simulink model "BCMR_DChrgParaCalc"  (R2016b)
settings: Solver=FixedStepDiscrete  StartTime=0.0  StopTime=10  FixedStep=0.01  RelTol=1e-3  EnableMultiTasking=on
undefined symbols (not defined in the file or in its folder): BCMR_ahDChgBattNominalCapa_C, BCMR_bCurrCalSelect_C, BCMR_bCurrIncDeltaLimEna_C, BCMR_bDChrgFulChkTenEna_C, BCMR_bDChrgFulChkThreeEna_C, BCMR_cntCoolDFC_CW, BCMR_cntSoh_CW, BCMR_G1E0PlatformSwPara_C, BCMR_iCurrDcr_C, BCMR_iDcChrgCurrAbnorm_T, BCMR_iDcChrgCurrAbnormMAP_T, BCMR_iDcChrgCurrNew_T, BCMR_iDcChrgCurrNewMAP_T, BCMR_iDcChrgCurrOld_T, BCMR_iDcChrgCurrOldAbnorm_T, BCMR_iDcChrgCurrOldAbnormMAP_T, BCMR_iDcChrgCurrOldMAP_T, BCMR_iDCCurrDecStep_C, BCMR_iDCCurrDecThrd_C, BCMR_iDCCurrDeltaLim_C, BCMR_iDCCurrDiff_C, BCMR_iDCCurrFil_C, BCMR_iDCCurrIncStep_C, BCMR_iDCCurrIncThrd_C, BCMR_iDChrgCurrCutOff_C, BCMR_kmAcmDist_C, BCMR_numCcsPwrSelc_C, BCMR_numCellVoltFull_C, BCMR_numCellVoltFullThree_C, BCMR_numCurrCalcEna, BCMR_pCcsPwrSelc_C, BCMR_pctBmsPwrRdc_C, BCMR_rCurrDcr_C, BCMR_rCurrIcr_C, BCMR_rDchrgLoadCoef_C, BCMR_tBattTempMaxFil_C, BCMR_tBattTempSelcLmtDwn_C, BCMR_tBattTempSelcLmtUp_C, BCMR_tDcChrgCellTemp1_A, BCMR_tDcChrgCellTemp2_A, BCMR_tDcChrgCellTemp_A, BCMR_tDchrgLoadLmt_C, BCMR_tiBattTempMaxFilDly_C, BCMR_tiBattTempSwitch_C, BCMR_tiCellVoltFullCnt_C, BCMR_tiCellVoltMaxFilDly_C, BCMR_tiCurrHysTimeDelay_C, BCMR_tiDcChrgPwrCCSDebs_C, BCMR_tiDChgFullPreHold_C, BCMR_tiDChrgCurrReqCalDly_C, BCMR_tiDChrgDetParaDebs_C, BCMR_tiDChrgFullBase_C, BCMR_tiDChrgFullDebs_C, BCMR_tiDChrgFulParaDebs_C, BCMR_tiDChrgFulWait_C, BCMR_tiDChrgParaBase_C, BCMR_tiHoldOnToCurrCalcOff_C, BCMR_tTempDisMapX_A, BCMR_tTempDisMapY_A, BCMR_uBattVoltOff_C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
libraries: simulink x34
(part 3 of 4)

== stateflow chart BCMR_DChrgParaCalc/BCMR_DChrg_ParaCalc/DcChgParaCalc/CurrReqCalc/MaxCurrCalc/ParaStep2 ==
  state Init
    en:
    ParaStep = 0;
  state ParaStep1
    en:
    ParaStep = BCMR_ParaStep_A[0];
  state ParaStep2
    en:
    ParaStep = BCMR_ParaStep_A[1];
  state ParaStep3
    en:
    ParaStep = BCMR_ParaStep_A[2];
  state ParaStep4
    en:
    ParaStep = BCMR_ParaStep_A[3];
  state ParaStep5
    en:
    ParaStep = BCMR_ParaStep_A[4];
  state ParaStep6
    en:
    ParaStep = BCMR_ParaStep_A[5];
  state ParaStep7
    en:
    ParaStep = BCMR_ParaStep_A[6];
  state ParaStep8
    en:
    ParaStep = BCMR_ParaStep_A[7];
  state ParaStep9
    en:
    ParaStep = BCMR_ParaStep_A[8];
  state ParaStep10
    en:
    ParaStep = BCMR_ParaStep_A[9];
  state ParaStep11
    en:
    ParaStep = BCMR_ParaStep_A[10];
  state ParaStep12
    en:
    ParaStep = BCMR_ParaStep_A[11];
  state ParaStep13
    en:
    ParaStep = BCMR_ParaStep_A[12];
  state ParaStep14
    en:
    ParaStep = BCMR_ParaStep_A[13];
  (default) -> Init
  Init -> (junction 26) : [BattTemp >= BCMR_BattPara_A[0]]
  (junction 488) -> Init
  (junction 26) -> (junction 27)
  (junction 489) -> (junction 488)
  Init -> ParaStep1 : [BattTemp < BCMR_BattPara_A[0]]
  (junction 453) -> ParaStep1
  (junction 456) -> (junction 453)
  ParaStep1 -> ParaStep2 : [BattTemp >= BCMR_BattPara_A[0] ]
  ParaStep2 -> (junction 456) : [BattTemp < BCMR_BattPara_A[0] ]
  (junction 27) -> ParaStep2
  (junction 447) -> (junction 456)
  (junction 27) -> (junction 28) : [BattTemp >= BCMR_BattPara_A[1] ]
  (junction 450) -> ParaStep2
  ParaStep2 -> ParaStep3 : [BattTemp >= BCMR_BattPara_A[1] ]
  (junction 444) -> (junction 450)
  (junction 28) -> ParaStep3
  ParaStep3 -> (junction 444) : [BattTemp < BCMR_BattPara_A[1] - BCMR_HysRng_C]
  (junction 444) -> (junction 447) : [BattTemp < BCMR_BattPara_A[0] ]
  (junction 28) -> (junction 29) : [BattTemp >= BCMR_BattPara_A[2] ]
  (junction 430) -> (junction 444)
  (junction 431) -> (junction 447)
  (junction 441) -> ParaStep3
  (junction 426) -> (junction 441)
  ParaStep3 -> ParaStep4 : [BattTemp >= BCMR_BattPara_A[2] ]
  ParaStep4 -> (junction 426) : [BattTemp < BCMR_BattPara_A[2] - BCMR_HysRng_C]
  (junction 426) -> (junction 430) : [BattTemp < BCMR_BattPara_A[1] - BCMR_HysRng_C]
  (junction 430) -> (junction 431) : [BattTemp < BCMR_BattPara_A[0] ]
  (junction 472) -> (junction 426)
  (junction 473) -> (junction 430)
  (junction 475) -> (junction 431)
  (junction 29) -> ParaStep4
  (junction 29) -> (junction 30) : [BattTemp >= BCMR_BattPara_A[3]]
  (junction 423) -> ParaStep4
  (junction 474) -> (junction 423)
  ParaStep4 -> ParaStep5 : [BattTemp >= BCMR_BattPara_A[3]]
  ParaStep5 -> (junction 474) : [BattTemp < BCMR_BattPara_A[3] - BCMR_HysRng_C]
  (junction 474) -> (junction 472) : [BattTemp < BCMR_BattPara_A[2] - BCMR_HysRng_C]
  (junction 472) -> (junction 473) : [BattTemp < BCMR_BattPara_A[1] - BCMR_HysRng_C]
  (junction 473) -> (junction 475) : [BattTemp < BCMR_BattPara_A[0] ]
  (junction 30) -> ParaStep5
  (junction 401) -> (junction 474)
  (junction 389) -> (junction 472)
  (junction 400) -> (junction 473)
  (junction 398) -> (junction 475)
  (junction 30) -> (junction 31) : [BattTemp >= BCMR_BattPara_A[4] ]
  (junction 408) -> ParaStep5
  (junction 392) -> (junction 408)
  ParaStep5 -> ParaStep6 : [BattTemp >= BCMR_BattPara_A[4] ]
  ParaStep6 -> (junction 392) : [BattTemp < BCMR_BattPara_A[4] - BCMR_HysRng_C]
  (junction 392) -> (junction 401) : [BattTemp < BCMR_BattPara_A[3] - BCMR_HysRng_C]
  (junction 401) -> (junction 389) : [BattTemp < BCMR_BattPara_A[2] - BCMR_HysRng_C]
  (junction 389) -> (junction 400) : [BattTemp < BCMR_BattPara_A[1] - BCMR_HysRng_C]
  (junction 400) -> (junction 398) : [BattTemp < BCMR_BattPara_A[0] ]
  (junction 375) -> (junction 392)
  (junction 371) -> (junction 401)
  (junction 364) -> (junction 389)
  (junction 369) -> (junction 400)
  (junction 376) -> (junction 398)
  (junction 31) -> ParaStep6
  (junction 31) -> (junction 74) : [BattTemp >= BCMR_BattPara_A[5] ]
  (junction 384) -> ParaStep6
  (junction 373) -> (junction 384)
  ParaStep6 -> ParaStep7 : [BattTemp >= BCMR_BattPara_A[5] ]
  ParaStep7 -> (junction 373) : [BattTemp < BCMR_BattPara_A[5] - BCMR_HysRng_C]
  (junction 373) -> (junction 375) : [BattTemp < BCMR_BattPara_A[4] - BCMR_HysRng_C]
  (junction 375) -> (junction 371) : [BattTemp < BCMR_BattPara_A[3] - BCMR_HysRng_C]
  (junction 371) -> (junction 364) : [BattTemp < BCMR_BattPara_A[2] - BCMR_HysRng_C]
  (junction 364) -> (junction 369) : [BattTemp < BCMR_BattPara_A[1] - BCMR_HysRng_C]
  (junction 369) -> (junction 376) : [BattTemp < BCMR_BattPara_A[0]]
  (junction 341) -> (junction 373)
  (junction 349) -> (junction 375)
  (junction 352) -> (junction 371)
  (junction 343) -> (junction 364)
  (junction 353) -> (junction 369)
  (junction 350) -> (junction 376)
  (junction 74) -> ParaStep7
  (junction 74) -> (junction 75) : [BattTemp >= BCMR_BattPara_A[6] ]
  (junction 169) -> ParaStep7
  (junction 337) -> (junction 169)
  ParaStep7 -> ParaStep8 : [BattTemp >= BCMR_BattPara_A[6] ]
  ParaStep8 -> (junction 337) : [BattTemp < BCMR_BattPara_A[6] - BCMR_HysRng_C]
  (junction 337) -> (junction 341) : [BattTemp < BCMR_BattPara_A[5] - BCMR_HysRng_C]
  (junction 341) -> (junction 349) : [BattTemp < BCMR_BattPara_A[4] - BCMR_HysRng_C]
  (junction 349) -> (junction 352) : [BattTemp < BCMR_BattPara_A[3] - BCMR_HysRng_C]
  (junction 352) -> (junction 343) : [BattTemp < BCMR_BattPara_A[2] - BCMR_HysRng_C]
  (junction 343) -> (junction 353) : [BattTemp < BCMR_BattPara_A[1] - BCMR_HysRng_C]
  (junction 353) -> (junction 350) : [BattTemp < BCMR_BattPara_A[0] ]
  (junction 75) -> ParaStep8
  (junction 313) -> (junction 337)
  (junction 321) -> (junction 341)
  (junction 328) -> (junction 349)
  (junction 331) -> (junction 352)
  (junction 319) -> (junction 343)
  (junction 334) -> (junction 353)
  (junction 330) -> (junction 350)
  (junction 75) -> (junction 76) : [BattTemp >= BCMR_BattPara_A[7] ]
  (junction 148) -> ParaStep8
  (junction 310) -> (junction 148)
  ParaStep8 -> ParaStep9 : [BattTemp >= BCMR_BattPara_A[7] ]
  ParaStep9 -> (junction 310) : [BattTemp < BCMR_BattPara_A[7] - BCMR_HysRng_C]
  (junction 310) -> (junction 313) : [BattTemp < BCMR_BattPara_A[6] - BCMR_HysRng_C]
  (junction 313) -> (junction 321) : [BattTemp < BCMR_BattPara_A[5] - BCMR_HysRng_C]
  (junction 321) -> (junction 328) : [BattTemp < BCMR_BattPara_A[4] - BCMR_HysRng_C]
  (junction 328) -> (junction 331) : [BattTemp < BCMR_BattPara_A[3] - BCMR_HysRng_C]
  (junction 331) -> (junction 319) : [BattTemp < BCMR_BattPara_A[2] - BCMR_HysRng_C]
  (junction 319) -> (junction 334) : [BattTemp < BCMR_BattPara_A[1] - BCMR_HysRng_C]
  (junction 334) -> (junction 330) : [BattTemp < BCMR_BattPara_A[0]]
  (junction 280) -> (junction 310)
  (junction 283) -> (junction 313)
  (junction 299) -> (junction 321)
  (junction 295) -> (junction 328)
  (junction 293) -> (junction 331)
  (junction 287) -> (junction 319)
  (junction 290) -> (junction 334)
  (junction 292) -> (junction 330)
  (junction 76) -> ParaStep9
  (junction 76) -> (junction 77) : [BattTemp >= BCMR_BattPara_A[8] ]
  (junction 140) -> ParaStep9
  (junction 277) -> (junction 140)
  ParaStep9 -> ParaStep10 : [BattTemp >= BCMR_BattPara_A[8] ]
  ParaStep10 -> (junction 277) : [BattTemp < BCMR_BattPara_A[8] - BCMR_HysRng_C]
  (junction 277) -> (junction 280) : [BattTemp < BCMR_BattPara_A[7] - BCMR_HysRng_C]
  (junction 280) -> (junction 283) : [BattTemp < BCMR_BattPara_A[6] - BCMR_HysRng_C]
  (junction 283) -> (junction 299) : [BattTemp < BCMR_BattPara_A[5] - BCMR_HysRng_C]
  (junction 299) -> (junction 295) : [BattTemp < BCMR_BattPara_A[4] - BCMR_HysRng_C]
  (junction 295) -> (junction 293) : [BattTemp < BCMR_BattPara_A[3] - BCMR_HysRng_C]
  (junction 293) -> (junction 287) : [BattTemp < BCMR_BattPara_A[2] - BCMR_HysRng_C]
  (junction 287) -> (junction 290) : [BattTemp < BCMR_BattPara_A[1] - BCMR_HysRng_C]
  (junction 290) -> (junction 292) : [BattTemp < BCMR_BattPara_A[0] ]
  (junction 228) -> (junction 277)
  (junction 230) -> (junction 280)
  (junction 232) -> (junction 283)
  (junction 247) -> (junction 299)
  (junction 253) -> (junction 295)
  (junction 249) -> (junction 293)
  (junction 259) -> (junction 287)
  (junction 256) -> (junction 290)
  (junction 246) -> (junction 292)
  (junction 77) -> ParaStep10
  (junction 77) -> (junction 78) : [BattTemp >= BCMR_BattPara_A[9] ]
  (junction 132) -> ParaStep10
  (junction 226) -> (junction 132)
  ParaStep10 -> ParaStep11 : [BattTemp >= BCMR_BattPara_A[9] ]
  ParaStep11 -> (junction 226) : [BattTemp < BCMR_BattPara_A[9] - BCMR_HysRng_C]
  (junction 226) -> (junction 228) : [BattTemp < BCMR_BattPara_A[8] - BCMR_HysRng_C]
  (junction 228) -> (junction 230) : [BattTemp < BCMR_BattPara_A[7] - BCMR_HysRng_C]
  (junction 230) -> (junction 232) : [BattTemp < BCMR_BattPara_A[6] - BCMR_HysRng_C]
  (junction 232) -> (junction 247) : [BattTemp < BCMR_BattPara_A[5] - BCMR_HysRng_C]
  (junction 247) -> (junction 253) : [BattTemp < BCMR_BattPara_A[4] - BCMR_HysRng_C]
  (junction 253) -> (junction 249) : [BattTemp < BCMR_BattPara_A[3] - BCMR_HysRng_C]
  (junction 249) -> (junction 259) : [BattTemp < BCMR_BattPara_A[2] - BCMR_HysRng_C]
  (junction 259) -> (junction 256) : [BattTemp < BCMR_BattPara_A[1] - BCMR_HysRng_C]
  (junction 256) -> (junction 246) : [BattTemp < BCMR_BattPara_A[0] ]
  (junction 78) -> ParaStep11
  (junction 196) -> (junction 226)
  (junction 199) -> (junction 228)
  (junction 202) -> (junction 230)
  (junction 205) -> (junction 232)
  (junction 213) -> (junction 247)
  (junction 210) -> (junction 253)
  (junction 211) -> (junction 249)
  (junction 212) -> (junction 259)
  (junction 222) -> (junction 256)
  (junction 220) -> (junction 246)
  (junction 78) -> (junction 79) : [BattTemp >= BCMR_BattPara_A[10]]
  (junction 127) -> ParaStep11
  (junction 241) -> (junction 127)
  ParaStep11 -> ParaStep12 : [BattTemp >= BCMR_BattPara_A[10]]
  ParaStep12 -> (junction 241) : [BattTemp < BCMR_BattPara_A[10] - BCMR_HysRng_C]
  (junction 241) -> (junction 196) : [BattTemp < BCMR_BattPara_A[9] - BCMR_HysRng_C]
  (junction 196) -> (junction 199) : [BattTemp < BCMR_BattPara_A[8] - BCMR_HysRng_C]
  (junction 199) -> (junction 202) : [BattTemp < BCMR_BattPara_A[7] - BCMR_HysRng_C]
  (junction 202) -> (junction 205) : [BattTemp < BCMR_BattPara_A[6] - BCMR_HysRng_C]
  (junction 205) -> (junction 213) : [BattTemp < BCMR_BattPara_A[5] - BCMR_HysRng_C]
  (junction 213) -> (junction 210) : [BattTemp < BCMR_BattPara_A[4] - BCMR_HysRng_C]
  (junction 210) -> (junction 211) : [BattTemp < BCMR_BattPara_A[3] - BCMR_HysRng_C]
  (junction 211) -> (junction 212) : [BattTemp < BCMR_BattPara_A[2] - BCMR_HysRng_C]
  (junction 212) -> (junction 222) : [BattTemp < BCMR_BattPara_A[1] - BCMR_HysRng_C]
  (junction 222) -> (junction 220) : [BattTemp < BCMR_BattPara_A[0] ]
  (junction 79) -> ParaStep12
  (junction 124) -> (junction 241)
  (junction 135) -> (junction 196)
  (junction 143) -> (junction 199)
  (junction 151) -> (junction 202)
  (junction 154) -> (junction 205)
  (junction 156) -> (junction 213)
  (junction 157) -> (junction 210)
  (junction 158) -> (junction 211)
  (junction 159) -> (junction 212)
  (junction 164) -> (junction 222)
  (junction 166) -> (junction 220)
  (junction 79) -> (junction 80) : [BattTemp >= BCMR_BattPara_A[11] ]
  (junction 119) -> ParaStep12
  (junction 238) -> (junction 119)
  ParaStep12 -> ParaStep13 : [BattTemp >= BCMR_BattPara_A[11] ]
  (junction 80) -> ParaStep13
  ParaStep13 -> (junction 238) : [BattTemp < BCMR_BattPara_A[11] - BCMR_HysRng_C]
  (junction 238) -> (junction 124) : [BattTemp < BCMR_BattPara_A[10] - BCMR_HysRng_C]
  (junction 124) -> (junction 135) : [BattTemp < BCMR_BattPara_A[9] - BCMR_HysRng_C]
  (junction 135) -> (junction 143) : [BattTemp < BCMR_BattPara_A[8] - BCMR_HysRng_C]
  (junction 143) -> (junction 151) : [BattTemp < BCMR_BattPara_A[7] - BCMR_HysRng_C]
  (junction 151) -> (junction 154) : [BattTemp < BCMR_BattPara_A[6] - BCMR_HysRng_C]
  (junction 154) -> (junction 156) : [BattTemp < BCMR_BattPara_A[5] - BCMR_HysRng_C]
  (junction 156) -> (junction 157) : [BattTemp < BCMR_BattPara_A[4] - BCMR_HysRng_C]
  (junction 157) -> (junction 158) : [BattTemp < BCMR_BattPara_A[3] - BCMR_HysRng_C]
  (junction 158) -> (junction 159) : [BattTemp < BCMR_BattPara_A[2] - BCMR_HysRng_C]
  (junction 159) -> (junction 164) : [BattTemp < BCMR_BattPara_A[1] - BCMR_HysRng_C]
  (junction 164) -> (junction 166) : [BattTemp < BCMR_BattPara_A[0] ]
  (junction 80) -> (junction 81) : [BattTemp >= BCMR_BattPara_A[12] ]
  (junction 115) -> (junction 238)
  (junction 117) -> (junction 124)
  (junction 130) -> (junction 135)
  (junction 138) -> (junction 143)
  (junction 146) -> (junction 151)
  (junction 181) -> (junction 154)
  (junction 179) -> (junction 156)
  (junction 176) -> (junction 157)
  (junction 177) -> (junction 158)
  (junction 178) -> (junction 159)
  (junction 185) -> (junction 164)
  (junction 184) -> (junction 166)
  (junction 462) -> ParaStep13
  (junction 460) -> (junction 462)
  ParaStep13 -> ParaStep14 : [BattTemp >= BCMR_BattPara_A[12] ]
  (junction 81) -> ParaStep14
  ParaStep14 -> (junction 460) : [BattTemp < BCMR_BattPara_A[12] - BCMR_HysRng_C]
  (junction 460) -> (junction 115) : [BattTemp < BCMR_BattPara_A[11] - BCMR_HysRng_C]
  (junction 115) -> (junction 117) : [BattTemp < BCMR_BattPara_A[10] - BCMR_HysRng_C]
  (junction 117) -> (junction 130) : [BattTemp < BCMR_BattPara_A[9] - BCMR_HysRng_C]
  (junction 130) -> (junction 138) : [BattTemp < BCMR_BattPara_A[8] - BCMR_HysRng_C]
  (junction 138) -> (junction 146) : [BattTemp < BCMR_BattPara_A[7] - BCMR_HysRng_C]
  (junction 146) -> (junction 181) : [BattTemp < BCMR_BattPara_A[6] - BCMR_HysRng_C]
  (junction 181) -> (junction 179) : [BattTemp < BCMR_BattPara_A[5] - BCMR_HysRng_C]
  (junction 179) -> (junction 176) : [BattTemp < BCMR_BattPara_A[4] - BCMR_HysRng_C]
  (junction 176) -> (junction 177) : [BattTemp < BCMR_BattPara_A[3] - BCMR_HysRng_C]
  (junction 177) -> (junction 178) : [BattTemp < BCMR_BattPara_A[2] - BCMR_HysRng_C]
  (junction 178) -> (junction 185) : [BattTemp < BCMR_BattPara_A[1] - BCMR_HysRng_C]
  (junction 185) -> (junction 184) : [BattTemp < BCMR_BattPara_A[0] ]
  (junction 81) -> (junction 467) : [BattTemp >= BCMR_BattPara_A[13] ]
  ParaStep14 -> (junction 493) : [BattTemp >= BCMR_BattPara_A[13] ]
  (junction 467) -> (junction 493)
  (junction 493) -> (junction 489)
  data: BattTemp input single; ParaStep output uint8; BCMR_BattPara_A input single; BCMR_ParaStep_A input uint8; BCMR_HysRng_C input single

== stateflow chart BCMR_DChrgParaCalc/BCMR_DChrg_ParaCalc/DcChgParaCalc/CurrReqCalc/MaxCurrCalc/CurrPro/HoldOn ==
  state Init
    en:
    CurrMethod = uint8(0);
  state HoldOn
    en:
    StepKeepL = VoltStepLast;
    StepKeepN = VoltStepNext;
    TempKeepL = TempStepL;
    TempKeepN = TempStep;
    CurrMethod = uint8(1);
  state CurrCalc
    state Init
      (default) -> (junction 296) : {CurrMethod = uint8(3);}
      (junction 296) -> (junction 297) : [FirstFlg == false]
      (junction 297) -> (junction 298) : [VoltStepFlg== true]
      (junction 296) -> (junction 301) : [FirstFlg == true] {CurrCalc = 0;}
      (junction 297) -> (junction 299)
      (junction 298) -> (junction 304) : {CurrCalc = CurrCalc; VoltStepFlg = false;}
      (junction 299) -> (junction 300) : [BCMR_bDChrgCoolAbnorm == true]
      (junction 299) -> (junction 302) : {CurrCalc = BCMR_iDcChrgCurrNew_T[TempKeepL][StepKeepL];}
      (junction 300) -> (junction 303) : {CurrCalc =  BCMR_iDcChrgCurrAbnorm_T[TempKeepL][StepKeepL];}
      (junction 302) -> (junction 301)
      (junction 303) -> (junction 302)
      (junction 304) -> (junction 303)
      (junction 301) -> (junction 305) : {CurrMethod = uint8(4);}
    state CurrSwitch
      (default) -> (junction 280)
      (junction 280) -> (junction 282) : [BCMR_bDChrgCoolAbnorm == true]
      (junction 280) -> (junction 281) : {CurrCompare = BCMR_iDcChrgCurrNew_T[TempKeepN][StepKeepN]; CurrMethod = uint8(5);}
      (junction 282) -> (junction 283) : {CurrCompare = BCMR_iDcChrgCurrAbnorm_T[TempKeepN][StepKeepN]; CurrMethod = uint8(6);}
      (junction 283) -> (junction 281)
      (junction 281) -> (junction 284)
    state CalcIcr
      en:
      CurrMethod = uint8(8);
      CurrCalc = CurrCalc + BCMR_rCurrIcr_C;
      du:
      CurrCalc = CurrCalc + BCMR_rCurrIcr_C;
    state CalcDcr
      en:
      CurrMethod = uint8(9);
      CurrCalc = CurrCalc - BCMR_rCurrDcr_C;
      du:
      CurrCalc = CurrCalc - BCMR_rCurrDcr_C;
    state End
      en:
      CurrMethod = uint8(10);
      TableChkFlg = true;
    (default) -> Init : {TableChkFlg = false;}
    Init -> CurrSwitch : [CurrMethod ==4]
    CurrSwitch -> CalcIcr : [(CurrCalc < CurrCompare) ]
    CurrSwitch -> CalcDcr : [(CurrCalc >= CurrCompare) ]
    CalcIcr -> End : [(CurrCalc >= CurrCompare) ] {FirstFlg = false;}
    CalcDcr -> End : [CurrCalc <= CurrCompare ]
  state ChkTable
    state Init
      en:
      CurrMethod = uint8(13);
    state Normal
      en:
      CurrMethod = uint8(14);
      CurrCalc = BCMR_iDcChrgCurrNew_T[TempStep][VoltStepNext];
    state Abnormal
      en:
      CurrMethod = uint8(15);
      CurrCalc = BCMR_iDcChrgCurrAbnorm_T[TempStep][VoltStepNext];
    (default) -> Init : {FirstFlg = false;}
    Init -> (junction 252) : [BCMR_bDChrgCoolAbnorm == true]
    (junction 252) -> (junction 253)
    Init -> Normal : [BCMR_bDChrgCoolAbnorm == false]
    (junction 253) -> Abnormal
  (default) -> Init : {FirstFlg = true;}
  Init -> HoldOn : [ VoltStepLast <= VoltStepNext ]
  (junction 267) -> HoldOn
  (junction 245) -> HoldOn
  (junction 265) -> (junction 267) : {FirstFlg = false; VoltStepFlg = true;}
  (junction 246) -> (junction 245)
  HoldOn -> CurrCalc : [after(BCMR_tiHoldOnToCurrCalc_C,sec)]
  CurrCalc -> (junction 265) : [VoltStepLast < VoltStepNext || TempStep ~= TempStepL]
  CurrCalc -> ChkTable : [TableChkFlg == true ]
  ChkTable -> (junction 246) : [ VoltStepLast < VoltStepNext || TempStep ~= TempStepL]
  data: VoltStepLast input uint8; CurrCalc output single; VoltStepNext input uint8; TempStep input uint8; StepKeepL local uint8; StepKeepN local uint8; TempStepL input uint8; FirstFlg local boolean; BCMR_rCurrDcr_C parameter single; CurrMethod output uint8; BCMR_bDChrgCoolAbnorm input boolean; BCMR_rCurrIcr_C parameter single; TableChkFlg local boolean; VoltStepFlg local boolean; CurrCompare local single; TempKeepL local uint8; TempKeepN local uint8; BCMR_iDcChrgCurrNew_T input single; BCMR_iDcChrgCurrAbnorm_T input single; BCMR_tiHoldOnToCurrCalc_C input single

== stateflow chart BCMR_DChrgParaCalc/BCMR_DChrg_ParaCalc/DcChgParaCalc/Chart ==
  state Store
    en:
    BCMR_rSocInit = BSER_rSoc;
  (default) -> Store
  data: BSER_rSoc input single; BCMR_rSocInit output single
  events: input RISING_EDGE_EVENT

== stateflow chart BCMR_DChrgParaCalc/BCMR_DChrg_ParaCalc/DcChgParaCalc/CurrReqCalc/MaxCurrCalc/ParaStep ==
  state Init
    en:
    ParaStep = 0;
  state ParaStep1
    en:
    ParaStep = BCMR_ParaStep_A[0];
  state ParaStep2
    en:
    ParaStep = BCMR_ParaStep_A[1];
  state ParaStep3
    en:
    ParaStep = BCMR_ParaStep_A[2];
  state ParaStep4
    en:
    ParaStep = BCMR_ParaStep_A[3];
  state ParaStep5
    en:
    ParaStep = BCMR_ParaStep_A[4];
  state ParaStep6
    en:
    ParaStep = BCMR_ParaStep_A[5];
  state ParaStep7
    en:
    ParaStep = BCMR_ParaStep_A[6];
  state ParaStep8
    en:
    ParaStep = BCMR_ParaStep_A[7];
  state ParaStep9
    en:
    ParaStep = BCMR_ParaStep_A[8];
  state ParaStep10
    en:
    ParaStep = BCMR_ParaStep_A[9];
  state ParaStep11
    en:
    ParaStep = BCMR_ParaStep_A[10];
  state ParaStep12
    en:
    ParaStep = BCMR_ParaStep_A[11];
  state ParaStep13
    en:
    ParaStep = BCMR_ParaStep_A[12];
  state ParaStep14
    en:
    ParaStep = BCMR_ParaStep_A[13];
  (default) -> Init
  Init -> (junction 26) : [BattTemp >= BCMR_BattPara_A[0]]
  (junction 488) -> Init
  (junction 26) -> (junction 27)
  (junction 489) -> (junction 488)
  Init -> ParaStep1 : [BattTemp < BCMR_BattPara_A[0] && after(3,sec)]
  (junction 453) -> ParaStep1
  (junction 456) -> (junction 453)
  ParaStep1 -> ParaStep2 : [BattTemp >= BCMR_BattPara_A[0] && after(BCMR_tiCurrHysTimeDelay_C,sec) ]
  ParaStep2 -> (junction 456) : [BattTemp < BCMR_BattPara_A[0] ]
  (junction 27) -> ParaStep2
  (junction 447) -> (junction 456)
  (junction 27) -> (junction 28) : [BattTemp >= BCMR_BattPara_A[1] ]
  (junction 450) -> ParaStep2
  ParaStep2 -> ParaStep3 : [BattTemp >= BCMR_BattPara_A[1] && after(BCMR_tiCurrHysTimeDelay_C,sec) ]
  (junction 444) -> (junction 450)
  (junction 28) -> ParaStep3
  ParaStep3 -> (junction 444) : [BattTemp < BCMR_BattPara_A[1] - BCMR_HysRng_C]
  (junction 444) -> (junction 447) : [BattTemp < BCMR_BattPara_A[0] ]
  (junction 28) -> (junction 29) : [BattTemp >= BCMR_BattPara_A[2] ]
  (junction 430) -> (junction 444)
  (junction 431) -> (junction 447)
  (junction 441) -> ParaStep3
  (junction 426) -> (junction 441)
  ParaStep3 -> ParaStep4 : [BattTemp >= BCMR_BattPara_A[2] && after(BCMR_tiCurrHysTimeDelay_C,sec) ]
  ParaStep4 -> (junction 426) : [BattTemp < BCMR_BattPara_A[2] - BCMR_HysRng_C]
  (junction 426) -> (junction 430) : [BattTemp < BCMR_BattPara_A[1] - BCMR_HysRng_C]
  (junction 430) -> (junction 431) : [BattTemp < BCMR_BattPara_A[0] ]
  (junction 472) -> (junction 426)
  (junction 473) -> (junction 430)
  (junction 475) -> (junction 431)
  (junction 29) -> ParaStep4
  (junction 29) -> (junction 30) : [BattTemp >= BCMR_BattPara_A[3]]
  (junction 423) -> ParaStep4
  (junction 474) -> (junction 423)
  ParaStep4 -> ParaStep5 : [BattTemp >= BCMR_BattPara_A[3] && after(BCMR_tiCurrHysTimeDelay_C,sec)]
  ParaStep5 -> (junction 474) : [BattTemp < BCMR_BattPara_A[3] - BCMR_HysRng_C]
  (junction 474) -> (junction 472) : [BattTemp < BCMR_BattPara_A[2] - BCMR_HysRng_C]
  (junction 472) -> (junction 473) : [BattTemp < BCMR_BattPara_A[1] - BCMR_HysRng_C]
  (junction 473) -> (junction 475) : [BattTemp < BCMR_BattPara_A[0] ]
  (junction 30) -> ParaStep5
  (junction 401) -> (junction 474)
  (junction 389) -> (junction 472)
  (junction 400) -> (junction 473)
  (junction 398) -> (junction 475)
  (junction 30) -> (junction 31) : [BattTemp >= BCMR_BattPara_A[4] ]
  (junction 408) -> ParaStep5
  (junction 392) -> (junction 408)
  ParaStep5 -> ParaStep6 : [BattTemp >= BCMR_BattPara_A[4] && after(BCMR_tiCurrHysTimeDelay_C,sec) ]
  ParaStep6 -> (junction 392) : [BattTemp < BCMR_BattPara_A[4] - BCMR_HysRng_C]
  (junction 392) -> (junction 401) : [BattTemp < BCMR_BattPara_A[3] - BCMR_HysRng_C]
  (junction 401) -> (junction 389) : [BattTemp < BCMR_BattPara_A[2] - BCMR_HysRng_C]
  (junction 389) -> (junction 400) : [BattTemp < BCMR_BattPara_A[1] - BCMR_HysRng_C]
  (junction 400) -> (junction 398) : [BattTemp < BCMR_BattPara_A[0] ]
  (junction 375) -> (junction 392)
  (junction 371) -> (junction 401)
  (junction 364) -> (junction 389)
  (junction 369) -> (junction 400)
  (junction 376) -> (junction 398)
  (junction 31) -> ParaStep6
  (junction 31) -> (junction 74) : [BattTemp >= BCMR_BattPara_A[5] ]
  (junction 384) -> ParaStep6
  (junction 373) -> (junction 384)
  ParaStep6 -> ParaStep7 : [BattTemp >= BCMR_BattPara_A[5] && after(BCMR_tiCurrHysTimeDelay_C,sec) ]
  ParaStep7 -> (junction 373) : [BattTemp < BCMR_BattPara_A[5] - BCMR_HysRng_C]
  (junction 373) -> (junction 375) : [BattTemp < BCMR_BattPara_A[4] - BCMR_HysRng_C]
  (junction 375) -> (junction 371) : [BattTemp < BCMR_BattPara_A[3] - BCMR_HysRng_C]
  (junction 371) -> (junction 364) : [BattTemp < BCMR_BattPara_A[2] - BCMR_HysRng_C]
  (junction 364) -> (junction 369) : [BattTemp < BCMR_BattPara_A[1] - BCMR_HysRng_C]
  (junction 369) -> (junction 376) : [BattTemp < BCMR_BattPara_A[0]]
  (junction 341) -> (junction 373)
  (junction 349) -> (junction 375)
  (junction 352) -> (junction 371)
  (junction 343) -> (junction 364)
  (junction 353) -> (junction 369)
  (junction 350) -> (junction 376)
  (junction 74) -> ParaStep7
  (junction 74) -> (junction 75) : [BattTemp >= BCMR_BattPara_A[6] ]
  (junction 169) -> ParaStep7
  (junction 337) -> (junction 169)
  ParaStep7 -> ParaStep8 : [BattTemp >= BCMR_BattPara_A[6] && after(BCMR_tiCurrHysTimeDelay_C,sec) ]
  ParaStep8 -> (junction 337) : [BattTemp < BCMR_BattPara_A[6] - BCMR_HysRng_C]
  (junction 337) -> (junction 341) : [BattTemp < BCMR_BattPara_A[5] - BCMR_HysRng_C]
  (junction 341) -> (junction 349) : [BattTemp < BCMR_BattPara_A[4] - BCMR_HysRng_C]
  (junction 349) -> (junction 352) : [BattTemp < BCMR_BattPara_A[3] - BCMR_HysRng_C]
  (junction 352) -> (junction 343) : [BattTemp < BCMR_BattPara_A[2] - BCMR_HysRng_C]
  (junction 343) -> (junction 353) : [BattTemp < BCMR_BattPara_A[1] - BCMR_HysRng_C]
  (junction 353) -> (junction 350) : [BattTemp < BCMR_BattPara_A[0] ]
  (junction 75) -> ParaStep8
  (junction 313) -> (junction 337)
  (junction 321) -> (junction 341)
  (junction 328) -> (junction 349)
  (junction 331) -> (junction 352)
  (junction 319) -> (junction 343)
  (junction 334) -> (junction 353)
  (junction 330) -> (junction 350)
  (junction 75) -> (junction 76) : [BattTemp >= BCMR_BattPara_A[7] ]
  (junction 148) -> ParaStep8
  (junction 310) -> (junction 148)
  ParaStep8 -> ParaStep9 : [BattTemp >= BCMR_BattPara_A[7] && after(BCMR_tiCurrHysTimeDelay_C,sec) ]
  ParaStep9 -> (junction 310) : [BattTemp < BCMR_BattPara_A[7] - BCMR_HysRng_C]
  (junction 310) -> (junction 313) : [BattTemp < BCMR_BattPara_A[6] - BCMR_HysRng_C]
  (junction 313) -> (junction 321) : [BattTemp < BCMR_BattPara_A[5] - BCMR_HysRng_C]
  (junction 321) -> (junction 328) : [BattTemp < BCMR_BattPara_A[4] - BCMR_HysRng_C]
  (junction 328) -> (junction 331) : [BattTemp < BCMR_BattPara_A[3] - BCMR_HysRng_C]
  (junction 331) -> (junction 319) : [BattTemp < BCMR_BattPara_A[2] - BCMR_HysRng_C]
  (junction 319) -> (junction 334) : [BattTemp < BCMR_BattPara_A[1] - BCMR_HysRng_C]
  (junction 334) -> (junction 330) : [BattTemp < BCMR_BattPara_A[0]]
  (junction 280) -> (junction 310)
  (junction 283) -> (junction 313)
  (junction 299) -> (junction 321)
  (junction 295) -> (junction 328)
  (junction 293) -> (junction 331)
  (junction 287) -> (junction 319)
  (junction 290) -> (junction 334)
  (junction 292) -> (junction 330)
  (junction 76) -> ParaStep9
  (junction 76) -> (junction 77) : [BattTemp >= BCMR_BattPara_A[8] ]
  (junction 140) -> ParaStep9
  (junction 277) -> (junction 140)
  ParaStep9 -> ParaStep10 : [BattTemp >= BCMR_BattPara_A[8] && after(BCMR_tiCurrHysTimeDelay_C,sec) ]
  ParaStep10 -> (junction 277) : [BattTemp < BCMR_BattPara_A[8] - BCMR_HysRng_C]
  (junction 277) -> (junction 280) : [BattTemp < BCMR_BattPara_A[7] - BCMR_HysRng_C]
  (junction 280) -> (junction 283) : [BattTemp < BCMR_BattPara_A[6] - BCMR_HysRng_C]
  (junction 283) -> (junction 299) : [BattTemp < BCMR_BattPara_A[5] - BCMR_HysRng_C]
  (junction 299) -> (junction 295) : [BattTemp < BCMR_BattPara_A[4] - BCMR_HysRng_C]
  (junction 295) -> (junction 293) : [BattTemp < BCMR_BattPara_A[3] - BCMR_HysRng_C]
  (junction 293) -> (junction 287) : [BattTemp < BCMR_BattPara_A[2] - BCMR_HysRng_C]
  (junction 287) -> (junction 290) : [BattTemp < BCMR_BattPara_A[1] - BCMR_HysRng_C]
  (junction 290) -> (junction 292) : [BattTemp < BCMR_BattPara_A[0] ]
  (junction 228) -> (junction 277)
  (junction 230) -> (junction 280)
  (junction 232) -> (junction 283)
  (junction 247) -> (junction 299)
  (junction 253) -> (junction 295)
  (junction 249) -> (junction 293)
  (junction 259) -> (junction 287)
  (junction 256) -> (junction 290)
  (junction 246) -> (junction 292)
  (junction 77) -> ParaStep10
  (junction 77) -> (junction 78) : [BattTemp >= BCMR_BattPara_A[9] ]
  (junction 132) -> ParaStep10
  (junction 226) -> (junction 132)
  ParaStep10 -> ParaStep11 : [BattTemp >= BCMR_BattPara_A[9] && after(BCMR_tiCurrHysTimeDelay_C,sec) ]
  ParaStep11 -> (junction 226) : [BattTemp < BCMR_BattPara_A[9] - BCMR_HysRng_C]
  (junction 226) -> (junction 228) : [BattTemp < BCMR_BattPara_A[8] - BCMR_HysRng_C]
  (junction 228) -> (junction 230) : [BattTemp < BCMR_BattPara_A[7] - BCMR_HysRng_C]
  (junction 230) -> (junction 232) : [BattTemp < BCMR_BattPara_A[6] - BCMR_HysRng_C]
  (junction 232) -> (junction 247) : [BattTemp < BCMR_BattPara_A[5] - BCMR_HysRng_C]
  (junction 247) -> (junction 253) : [BattTemp < BCMR_BattPara_A[4] - BCMR_HysRng_C]
  (junction 253) -> (junction 249) : [BattTemp < BCMR_BattPara_A[3] - BCMR_HysRng_C]
  (junction 249) -> (junction 259) : [BattTemp < BCMR_BattPara_A[2] - BCMR_HysRng_C]
  (junction 259) -> (junction 256) : [BattTemp < BCMR_BattPara_A[1] - BCMR_HysRng_C]
  (junction 256) -> (junction 246) : [BattTemp < BCMR_BattPara_A[0] ]
  (junction 78) -> ParaStep11
  (junction 196) -> (junction 226)
  (junction 199) -> (junction 228)
  (junction 202) -> (junction 230)
  (junction 205) -> (junction 232)
  (junction 213) -> (junction 247)
  (junction 210) -> (junction 253)
  (junction 211) -> (junction 249)
  (junction 212) -> (junction 259)
  (junction 222) -> (junction 256)
  (junction 220) -> (junction 246)
  (junction 78) -> (junction 79) : [BattTemp >= BCMR_BattPara_A[10]]
  (junction 127) -> ParaStep11
  (junction 241) -> (junction 127)
  ParaStep11 -> ParaStep12 : [BattTemp >= BCMR_BattPara_A[10] && after(BCMR_tiCurrHysTimeDelay_C,sec)]
  ParaStep12 -> (junction 241) : [BattTemp < BCMR_BattPara_A[10] - BCMR_HysRng_C]
  (junction 241) -> (junction 196) : [BattTemp < BCMR_BattPara_A[9] - BCMR_HysRng_C]
  (junction 196) -> (junction 199) : [BattTemp < BCMR_BattPara_A[8] - BCMR_HysRng_C]
  (junction 199) -> (junction 202) : [BattTemp < BCMR_BattPara_A[7] - BCMR_HysRng_C]
  (junction 202) -> (junction 205) : [BattTemp < BCMR_BattPara_A[6] - BCMR_HysRng_C]
  (junction 205) -> (junction 213) : [BattTemp < BCMR_BattPara_A[5] - BCMR_HysRng_C]
  (junction 213) -> (junction 210) : [BattTemp < BCMR_BattPara_A[4] - BCMR_HysRng_C]
  (junction 210) -> (junction 211) : [BattTemp < BCMR_BattPara_A[3] - BCMR_HysRng_C]
  (junction 211) -> (junction 212) : [BattTemp < BCMR_BattPara_A[2] - BCMR_HysRng_C]
  (junction 212) -> (junction 222) : [BattTemp < BCMR_BattPara_A[1] - BCMR_HysRng_C]
  (junction 222) -> (junction 220) : [BattTemp < BCMR_BattPara_A[0] ]
  (junction 79) -> ParaStep12
  (junction 124) -> (junction 241)
  (junction 135) -> (junction 196)
  (junction 143) -> (junction 199)
  (junction 151) -> (junction 202)
  (junction 154) -> (junction 205)
  (junction 156) -> (junction 213)
  (junction 157) -> (junction 210)
  (junction 158) -> (junction 211)
  (junction 159) -> (junction 212)
  (junction 164) -> (junction 222)
  (junction 166) -> (junction 220)
  (junction 79) -> (junction 80) : [BattTemp >= BCMR_BattPara_A[11] ]
  (junction 119) -> ParaStep12
  (junction 238) -> (junction 119)
  ParaStep12 -> ParaStep13 : [BattTemp >= BCMR_BattPara_A[11] && after(BCMR_tiCurrHysTimeDelay_C,sec) ]
  (junction 80) -> ParaStep13
  ParaStep13 -> (junction 238) : [BattTemp < BCMR_BattPara_A[11] - BCMR_HysRng_C]
  (junction 238) -> (junction 124) : [BattTemp < BCMR_BattPara_A[10] - BCMR_HysRng_C]
  (junction 124) -> (junction 135) : [BattTemp < BCMR_BattPara_A[9] - BCMR_HysRng_C]
  (junction 135) -> (junction 143) : [BattTemp < BCMR_BattPara_A[8] - BCMR_HysRng_C]
  (junction 143) -> (junction 151) : [BattTemp < BCMR_BattPara_A[7] - BCMR_HysRng_C]
  (junction 151) -> (junction 154) : [BattTemp < BCMR_BattPara_A[6] - BCMR_HysRng_C]
  (junction 154) -> (junction 156) : [BattTemp < BCMR_BattPara_A[5] - BCMR_HysRng_C]
  (junction 156) -> (junction 157) : [BattTemp < BCMR_BattPara_A[4] - BCMR_HysRng_C]
  (junction 157) -> (junction 158) : [BattTemp < BCMR_BattPara_A[3] - BCMR_HysRng_C]
  (junction 158) -> (junction 159) : [BattTemp < BCMR_BattPara_A[2] - BCMR_HysRng_C]
  (junction 159) -> (junction 164) : [BattTemp < BCMR_BattPara_A[1] - BCMR_HysRng_C]
  (junction 164) -> (junction 166) : [BattTemp < BCMR_BattPara_A[0] ]
  (junction 80) -> (junction 81) : [BattTemp >= BCMR_BattPara_A[12] ]
  (junction 115) -> (junction 238)
  (junction 117) -> (junction 124)
  (junction 130) -> (junction 135)
  (junction 138) -> (junction 143)
  (junction 146) -> (junction 151)
  (junction 181) -> (junction 154)
  (junction 179) -> (junction 156)
  (junction 176) -> (junction 157)
  (junction 177) -> (junction 158)
  (junction 178) -> (junction 159)
  (junction 185) -> (junction 164)
  (junction 184) -> (junction 166) : [after(BCMR_tiDChrgFulWait_C,sec)]
  (junction 462) -> ParaStep13
  (junction 460) -> (junction 462)
  ParaStep13 -> ParaStep14 : [BattTemp >= BCMR_BattPara_A[12] && after(BCMR_tiCurrHysTimeDelay_C,sec) ]
  (junction 81) -> ParaStep14
  ParaStep14 -> (junction 460) : [BattTemp < BCMR_BattPara_A[12] - BCMR_HysRng_C]
  (junction 460) -> (junction 115) : [BattTemp < BCMR_BattPara_A[11] - BCMR_HysRng_C]
  (junction 115) -> (junction 117) : [BattTemp < BCMR_BattPara_A[10] - BCMR_HysRng_C]
  (junction 117) -> (junction 130) : [BattTemp < BCMR_BattPara_A[9] - BCMR_HysRng_C]
  (junction 130) -> (junction 138) : [BattTemp < BCMR_BattPara_A[8] - BCMR_HysRng_C]
  (junction 138) -> (junction 146) : [BattTemp < BCMR_BattPara_A[7] - BCMR_HysRng_C]
  (junction 146) -> (junction 181) : [BattTemp < BCMR_BattPara_A[6] - BCMR_HysRng_C]
  (junction 181) -> (junction 179) : [BattTemp < BCMR_BattPara_A[5] - BCMR_HysRng_C]
  (junction 179) -> (junction 176) : [BattTemp < BCMR_BattPara_A[4] - BCMR_HysRng_C]
  (junction 176) -> (junction 177) : [BattTemp < BCMR_BattPara_A[3] - BCMR_HysRng_C]
  (junction 177) -> (junction 178) : [BattTemp < BCMR_BattPara_A[2] - BCMR_HysRng_C]
  (junction 178) -> (junction 185) : [BattTemp < BCMR_BattPara_A[1] - BCMR_HysRng_C]
  (junction 185) -> (junction 184) : [BattTemp < BCMR_BattPara_A[0] ]
  (junction 81) -> (junction 467) : [BattTemp >= BCMR_BattPara_A[13] && after(BCMR_tiDChrgFulWait_C,sec)]
  ParaStep14 -> (junction 493) : [BattTemp >= BCMR_BattPara_A[13] && (after(BCMR_tiDChrgFulWait_C,sec) && BCMR_flgDChrgFulChk == true)]
  (junction 467) -> (junction 493)
  (junction 493) -> (junction 489)
  data: BattTemp input single; ParaStep output uint8; BCMR_BattPara_A input single; BCMR_ParaStep_A input uint8; BCMR_HysRng_C input single; BCMR_tiDChrgFulWait_C parameter single; BCMR_flgDChrgFulChk input boolean; BCMR_tiCurrHysTimeDelay_C parameter single

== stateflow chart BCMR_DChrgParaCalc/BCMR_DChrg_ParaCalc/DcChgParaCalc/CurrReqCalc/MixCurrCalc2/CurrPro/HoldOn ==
  state Init
    en:
    CurrMethod = uint8(0);
  state HoldOn
    en:
    StepKeepL = VoltStepLast;
    StepKeepN = VoltStepNext;
    TempKeepL = TempStepL;
    TempKeepN = TempStep;
    CurrMethod = uint8(1);
  state CurrCalc
    state Init
      (default) -> (junction 296) : {CurrMethod = uint8(3);}
      (junction 296) -> (junction 297) : [FirstFlg == false]
      (junction 297) -> (junction 298) : [VoltStepFlg== true]
      (junction 296) -> (junction 301) : [FirstFlg == true] {CurrCalc = 0;}
      (junction 297) -> (junction 299)
      (junction 298) -> (junction 304) : {CurrCalc = CurrCalc; VoltStepFlg = false;}
      (junction 299) -> (junction 300) : [BCMR_bDChrgCoolAbnorm == true]
      (junction 299) -> (junction 302) : {CurrCalc = BCMR_iDcChrgCurrNew_T[TempKeepL][StepKeepL];}
      (junction 300) -> (junction 303) : {CurrCalc =  BCMR_iDcChrgCurrAbnorm_T[TempKeepL][StepKeepL];}
      (junction 302) -> (junction 301)
      (junction 303) -> (junction 302)
      (junction 304) -> (junction 303)
      (junction 301) -> (junction 305) : {CurrMethod = uint8(4);}
    state CurrSwitch
      (default) -> (junction 280)
      (junction 280) -> (junction 282) : [BCMR_bDChrgCoolAbnorm == true]
      (junction 280) -> (junction 281) : {CurrCompare = BCMR_iDcChrgCurrNew_T[TempKeepN][StepKeepN]; CurrMethod = uint8(5);}
      (junction 282) -> (junction 283) : {CurrCompare = BCMR_iDcChrgCurrAbnorm_T[TempKeepN][StepKeepN]; CurrMethod = uint8(6);}
      (junction 283) -> (junction 281)
      (junction 281) -> (junction 284)
    state CalcIcr
      en:
      CurrMethod = uint8(8);
      CurrCalc = CurrCalc + BCMR_rCurrIcr_C;
      du:
      CurrCalc = CurrCalc + BCMR_rCurrIcr_C;
    state CalcDcr
      en:
      CurrMethod = uint8(9);
      CurrCalc = CurrCalc - BCMR_rCurrDcr_C;
      du:
      CurrCalc = CurrCalc - BCMR_rCurrDcr_C;
    state End
      en:
      CurrMethod = uint8(10);
      TableChkFlg = true;
    (default) -> Init : {TableChkFlg = false;}
    Init -> CurrSwitch : [CurrMethod ==4]
    CurrSwitch -> CalcIcr : [(CurrCalc < CurrCompare) ]
    CurrSwitch -> CalcDcr : [(CurrCalc >= CurrCompare) ]
    CalcIcr -> End : [(CurrCalc >= CurrCompare) ] {FirstFlg = false;}
    CalcDcr -> End : [CurrCalc <= CurrCompare ]
  state ChkTable
    state Init
      en:
      CurrMethod = uint8(13);
    state Normal
      en:
      CurrMethod = uint8(14);
      CurrCalc = BCMR_iDcChrgCurrNew_T[TempStep][VoltStepNext];
    state Abnormal
      en:
      CurrMethod = uint8(15);
      CurrCalc = BCMR_iDcChrgCurrAbnorm_T[TempStep][VoltStepNext];
    (default) -> Init : {FirstFlg = false;}
    Init -> (junction 252) : [BCMR_bDChrgCoolAbnorm == true]
    (junction 252) -> (junction 253)
    Init -> Normal : [BCMR_bDChrgCoolAbnorm == false]
    (junction 253) -> Abnormal
  (default) -> Init : {FirstFlg = true;}
  Init -> HoldOn : [ VoltStepLast <= VoltStepNext ]
  (junction 267) -> HoldOn
  (junction 245) -> HoldOn
  (junction 265) -> (junction 267) : {FirstFlg = false; VoltStepFlg = true;}
  (junction 246) -> (junction 245)
  HoldOn -> CurrCalc : [after(BCMR_tiHoldOnToCurrCalc_C,sec)]
  CurrCalc -> (junction 265) : [VoltStepLast < VoltStepNext || TempStep ~= TempStepL]
  CurrCalc -> ChkTable : [TableChkFlg == true ]
  ChkTable -> (junction 246) : [ VoltStepLast < VoltStepNext || TempStep ~= TempStepL]
  data: VoltStepLast input uint8; CurrCalc output single; VoltStepNext input uint8; TempStep input uint8; StepKeepL local uint8; StepKeepN local uint8; TempStepL input uint8; FirstFlg local boolean; BCMR_rCurrDcr_C parameter single; CurrMethod output uint8; BCMR_bDChrgCoolAbnorm input boolean; BCMR_rCurrIcr_C parameter single; TableChkFlg local boolean; VoltStepFlg local boolean; CurrCompare local single; TempKeepL local uint8; TempKeepN local uint8; BCMR_iDcChrgCurrNew_T input single; BCMR_iDcChrgCurrAbnorm_T input single; BCMR_tiHoldOnToCurrCalc_C input single
